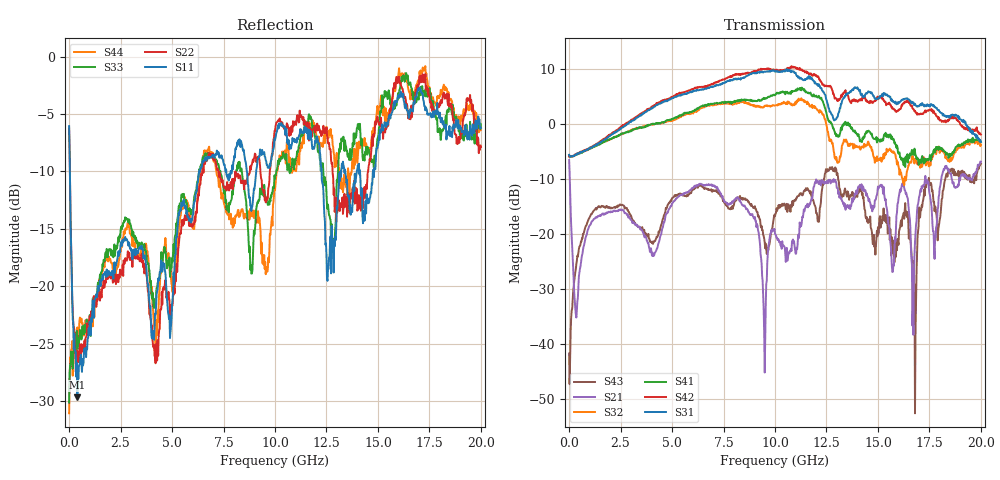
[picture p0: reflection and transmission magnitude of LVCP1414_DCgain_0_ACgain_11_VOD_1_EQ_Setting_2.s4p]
!Agilent Technologies,N5230A,MY46400459,A.07.50.48
!Agilent N5230A: A.07.50.48
!Date: Tuesday, April 17, 2012 18:30:07
!Correction: S11(Full 4 Port(1,2,3,4))
!S12(Full 4 Port(1,2,3,4))
!S13(Full 4 Port(1,2,3,4))
!S14(Full 4 Port(1,2,3,4))
!S21(Full 4 Port(1,2,3,4))
!S22(Full 4 Port(1,2,3,4))
!S23(Full 4 Port(1,2,3,4))
!S24(Full 4 Port(1,2,3,4))
!S31(Full 4 Port(1,2,3,4))
!S32(Full 4 Port(1,2,3,4))
!S33(Full 4 Port(1,2,3,4))
!S34(Full 4 Port(1,2,3,4))
!S41(Full 4 Port(1,2,3,4))
!S42(Full 4 Port(1,2,3,4))
!S43(Full 4 Port(1,2,3,4))
!S44(Full 4 Port(1,2,3,4))
!S4P File: Measurements: <S11,S12,S13,S14>,
!<S21,S22,S23,S24>,
!<S31,S32,S33,S34>,
!<S41,S42,S43,S44>:
# Hz S  dB  R 50
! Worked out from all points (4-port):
!   801 points, 300 kHz to 20 GHz, reference 50 ohm
!   strongest paths, dB at 300 kHz, 5 GHz, 10 GHz, 15 GHz, 20 GHz:
!     S31: -5.6, 4.7, 9.6, 4.6, -3.2
!     S42: -5.9, 5.0, 9.8, 4.9, -1.9
!     S41: -5.6, 1.0, 5.3, -2.6, -3.2
!     S32: -5.8, 0.7, 3.4, -6.6, -3.7
!     S21: -6.5, -14.4, -19.9, -11.3, -6.8
!     S43: -41.7, -13.4, -16.7, -18.7, -7.2
!   lowest |S11| = -29.7 dB at 400.3 MHz (marker M1), VSWR 1.07, Z = 53 + j1.46 ohm
!   |S11| at or under -10 dB: 37.33 MHz to 6.319 GHz (6.282 GHz wide, 198 % of centre); 12.26 GHz to 13.22 GHz (957.5 MHz wide, 7.52 % of centre); 14.13 GHz to 14.76 GHz (632 MHz wide, 4.38 % of centre)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
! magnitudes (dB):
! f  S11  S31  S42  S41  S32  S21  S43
! 300 kHz  -6.1  -5.6  -5.9  -5.6  -5.8  -6.5  -41.7
! 400.3 MHz  -29.7  -5.3  -5.3  -5.4  -5.4  -32.3  -23.9
! 10.08 GHz  -6.6  9.7  10.0  5.7  3.5  -20.7  -15.3
! 12.75 GHz  -14.7  1.8  6.5  0.1  -3.2  -10.5  -8.1
! 16.78 GHz  -4.1  3.7  2.4  -4.4  -7.1  -23.8  -29.1
! 17.4 GHz  -5.0  3.6  2.5  -6.6  -6.6  -10.2  -10.4
! 20 GHz  -6.2  -3.2  -1.9  -3.2  -3.7  -6.8  -7.2
